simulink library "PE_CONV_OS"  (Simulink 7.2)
settings: Solver=ode45  SolverMode=SingleTasking  StartTime=0.0  StopTime=10.0  RelTol=1e-3
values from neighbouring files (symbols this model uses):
  C = 10e-3*1    (= 0.01)    [INIT_B6_2L_3Ph_IGBT_OS.m]    (also in INIT_B6_3L_3Ph_IGBT_OS.m; INIT_MMC_100L.m = 0.005; INIT_MMC_200L.m = 0.005; INIT_MMC_20L.m)
  FS = 900    [INIT_B6_2L_3Ph_IGBT_OS.m]    (also in INIT_B6_3L_3Ph_IGBT_OS.m; INIT_PWM_2L.m = 1000; INIT_PWM_3L.m = 1000; INIT_PWM_Con.m = 1000)
  LN = 2e-3    (= 0.002)    [INIT_PWM_2L.m]    (also in INIT_PWM_3L.m; INIT_PWM_Con.m; INIT_MMC_100L.m = 0.025; INIT_MMC_200L.m = 0.025)
  LS = 1e-3    (= 0.001)    [INIT_B6_2L_3Ph_IGBT_OS.m]    (also in INIT_B6_3L_3Ph_IGBT_OS.m; INIT_MMC_100L.m = 0.025; INIT_MMC_200L.m = 0.025; INIT_MMC_20L.m = 0.0025)
  LT = LN    (= 0.025)    [INIT_MMC_100L.m]    (also in INIT_MMC_200L.m; INIT_MMC_20L.m = 0.002; INIT_MMC_400L.m)
  Nc = 100    [INIT_MMC_100L.m]    (also in INIT_MMC_200L.m = 200; INIT_MMC_20L.m = 20; INIT_MMC_400L.m = 400)
  NT = sqrt(3)*340/400    [INIT_MMC_100L.m]    (also in INIT_MMC_200L.m; INIT_MMC_20L.m = sqrt(3); INIT_MMC_400L.m)
  Rg = 1e-3    (= 0.001)    [INIT_MMC_100L.m]    (also in INIT_MMC_200L.m; INIT_MMC_20L.m; INIT_MMC_400L.m)
  RN = 0.1    [INIT_PWM_2L.m]    (also in INIT_PWM_3L.m; INIT_PWM_Con.m; INIT_MMC_100L.m; INIT_MMC_200L.m)
  RT = RN    (= 0.1)    [INIT_MMC_100L.m]    (also in INIT_MMC_200L.m; INIT_MMC_20L.m; INIT_MMC_400L.m)
  UC0 = 600    [INIT_B6_2L_3Ph_IGBT_OS.m]    (also in INIT_B6_3L_3Ph_IGBT_OS.m = 500; INIT_MMC_100L.m = 6800; INIT_MMC_200L.m = 3400; INIT_MMC_20L.m = 5000)
undefined symbols (not defined in the file or in its folder): A, DT, FT, L, O1, O2, PHT, T, Td
libraries: simulink_extras x2
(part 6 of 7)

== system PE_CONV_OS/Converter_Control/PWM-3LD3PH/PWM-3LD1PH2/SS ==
  I1 : Inport  OutDataType=sfix(16)  OutScaling=2^0
  DT : DataTypeConversion
  DT1 : DataTypeConversion
  Relay : Relay  OutDataType=sfix(16)  OutScaling=2^0
  Sum : Sum  Inputs=+-  OutDataType=sfix(16)  OutScaling=2^0
  TonDelay : Subsystem  mask(TonDelay){DT=DT}
      mask prompts: DT "Dead Time"
      mask help: Turn on dead time to protect against short circuit of the converter leg
  TonDelay1 : Subsystem  mask(TonDelay){DT=DT}
      mask prompts: DT "Dead Time"
      mask help: Turn on dead time to protect against short circuit of the converter leg
  TriGtr-AO : Subsystem  mask(TriGtr-AO){A=A, O=O1, T=1/FT, Td=PHT/FT/180}
      mask prompts: A "Amplitude"; O "Offset"; T "Period Time"; Td "Time Delay"
      mask help: Triangular Wave Generator with variable time delay, variable amplitude and offset
  not : Logic  Operator=NOT  Inputs=1
  O1 : Outport  InitialOutput=0
  O2 : Outport  Port=2  InitialOutput=0
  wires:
  DT1/1 -> not/1
  DT/1 -> TonDelay1/1(s1)
  I1/1 -> Sum/1
  TriGtr-AO/1(Out1) -> Sum/2
  Sum/1 -> Relay/1
  not/1 -> DT/1
  TonDelay1/1(s1d) -> O2/1
  Relay/1 -> DT1/1, TonDelay/1(s1)
  TonDelay/1(s1d) -> O1/1

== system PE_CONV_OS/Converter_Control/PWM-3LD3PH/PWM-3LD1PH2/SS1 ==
  I1 : Inport  OutDataType=sfix(16)  OutScaling=2^0
  DT : DataTypeConversion
  DT1 : DataTypeConversion
  Relay : Relay  OutDataType=sfix(16)  OutScaling=2^0
  Sum : Sum  Inputs=+-  OutDataType=sfix(16)  OutScaling=2^0
  TonDelay : Subsystem  mask(TonDelay){DT=DT}
      mask prompts: DT "Dead Time"
      mask help: Turn on dead time to protect against short circuit of the converter leg
  TonDelay1 : Subsystem  mask(TonDelay){DT=DT}
      mask prompts: DT "Dead Time"
      mask help: Turn on dead time to protect against short circuit of the converter leg
  TriGtr-AO : Subsystem  mask(TriGtr-AO){A=A, O=O2, T=1/FT, Td=PHT/FT/180}
      mask prompts: A "Amplitude"; O "Offset"; T "Period Time"; Td "Time Delay"
      mask help: Triangular Wave Generator with variable time delay, variable amplitude and offset
  not : Logic  Operator=NOT  Inputs=1
  O1 : Outport  InitialOutput=0
  O2 : Outport  Port=2  InitialOutput=0
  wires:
  DT1/1 -> not/1
  DT/1 -> TonDelay1/1(s1)
  I1/1 -> Sum/1
  TriGtr-AO/1(Out1) -> Sum/2
  Sum/1 -> Relay/1
  not/1 -> DT/1
  TonDelay1/1(s1d) -> O2/1
  Relay/1 -> DT1/1, TonDelay/1(s1)
  TonDelay/1(s1d) -> O1/1

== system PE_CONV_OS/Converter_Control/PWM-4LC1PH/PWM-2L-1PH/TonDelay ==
  s1 : Inport  Orientation=down  OutDataType=sfix(16)  OutScaling=2^0
  Int : Integrator  ExternalReset=falling
  Rel1 : Relay  OnSwitchValue=DT  OutDataType=sfix(16)  OutScaling=2^0
  s1d : Outport  InitialOutput=0
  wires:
  Rel1/1 -> s1d/1
  s1/1 -> Int/1, Int/2
  Int/1 -> Rel1/1

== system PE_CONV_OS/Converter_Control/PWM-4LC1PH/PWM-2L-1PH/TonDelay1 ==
  s1 : Inport  Orientation=down  OutDataType=sfix(16)  OutScaling=2^0
  Int : Integrator  ExternalReset=falling
  Rel1 : Relay  OnSwitchValue=DT  OutDataType=sfix(16)  OutScaling=2^0
  s1d : Outport  InitialOutput=0
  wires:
  Rel1/1 -> s1d/1
  s1/1 -> Int/1, Int/2
  Int/1 -> Rel1/1

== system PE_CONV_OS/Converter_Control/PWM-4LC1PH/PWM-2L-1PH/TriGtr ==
  Clock : Clock
  S1 : Subsystem
  Sum : Sum  OutDataType=sfix(16)  OutScaling=2^0
  T : Constant  Value=T  OutDataType=sfix(16)  OutScaling=2^0
  Td : Constant  Value=Td  OutDataType=sfix(16)  OutScaling=2^0
  mod : Math  Operator=mod
  O : Outport  InitialOutput=0
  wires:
  Td/1 -> Sum/2
  Sum/1 -> mod/1
  T/1 -> mod/2
  Clock/1 -> Sum/1
  S1/1(Out1) -> O/1
  mod/1 -> S1/1(In1)

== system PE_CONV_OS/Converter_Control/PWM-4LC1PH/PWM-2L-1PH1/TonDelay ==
  s1 : Inport  Orientation=down  OutDataType=sfix(16)  OutScaling=2^0
  Int : Integrator  ExternalReset=falling
  Rel1 : Relay  OnSwitchValue=DT  OutDataType=sfix(16)  OutScaling=2^0
  s1d : Outport  InitialOutput=0
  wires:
  Int/1 -> Rel1/1
  s1/1 -> Int/2, Int/1
  Rel1/1 -> s1d/1

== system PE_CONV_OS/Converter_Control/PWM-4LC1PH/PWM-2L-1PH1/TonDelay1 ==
  s1 : Inport  Orientation=down  OutDataType=sfix(16)  OutScaling=2^0
  Int : Integrator  ExternalReset=falling
  Rel1 : Relay  OnSwitchValue=DT  OutDataType=sfix(16)  OutScaling=2^0
  s1d : Outport  InitialOutput=0
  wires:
  Int/1 -> Rel1/1
  s1/1 -> Int/2, Int/1
  Rel1/1 -> s1d/1

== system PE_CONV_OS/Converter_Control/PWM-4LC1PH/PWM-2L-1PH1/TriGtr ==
  Clock : Clock
  S1 : Subsystem
  Sum : Sum  OutDataType=sfix(16)  OutScaling=2^0
  T : Constant  Value=T  OutDataType=sfix(16)  OutScaling=2^0
  Td : Constant  Value=Td  OutDataType=sfix(16)  OutScaling=2^0
  mod : Math  Operator=mod
  O : Outport  InitialOutput=0
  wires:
  mod/1 -> S1/1(In1)
  S1/1(Out1) -> O/1
  Clock/1 -> Sum/1
  T/1 -> mod/2
  Sum/1 -> mod/1
  Td/1 -> Sum/2

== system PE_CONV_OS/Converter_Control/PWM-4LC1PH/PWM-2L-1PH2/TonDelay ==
  s1 : Inport  Orientation=down  OutDataType=sfix(16)  OutScaling=2^0
  Int : Integrator  ExternalReset=falling
  Rel1 : Relay  OnSwitchValue=DT  OutDataType=sfix(16)  OutScaling=2^0
  s1d : Outport  InitialOutput=0
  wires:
  Rel1/1 -> s1d/1
  s1/1 -> Int/1, Int/2
  Int/1 -> Rel1/1

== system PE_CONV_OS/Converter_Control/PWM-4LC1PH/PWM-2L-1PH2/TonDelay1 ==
  s1 : Inport  Orientation=down  OutDataType=sfix(16)  OutScaling=2^0
  Int : Integrator  ExternalReset=falling
  Rel1 : Relay  OnSwitchValue=DT  OutDataType=sfix(16)  OutScaling=2^0
  s1d : Outport  InitialOutput=0
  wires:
  Rel1/1 -> s1d/1
  s1/1 -> Int/1, Int/2
  Int/1 -> Rel1/1

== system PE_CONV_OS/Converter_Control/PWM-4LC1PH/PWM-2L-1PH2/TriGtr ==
  Clock : Clock
  S1 : Subsystem
  Sum : Sum  OutDataType=sfix(16)  OutScaling=2^0
  T : Constant  Value=T  OutDataType=sfix(16)  OutScaling=2^0
  Td : Constant  Value=Td  OutDataType=sfix(16)  OutScaling=2^0
  mod : Math  Operator=mod
  O : Outport  InitialOutput=0
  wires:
  Td/1 -> Sum/2
  Sum/1 -> mod/1
  T/1 -> mod/2
  Clock/1 -> Sum/1
  S1/1(Out1) -> O/1
  mod/1 -> S1/1(In1)

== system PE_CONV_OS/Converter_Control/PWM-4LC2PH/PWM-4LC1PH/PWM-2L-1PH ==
  In1 : Inport  OutDataType=sfix(16)  OutScaling=2^0
  DT : DataTypeConversion
  DT1 : DataTypeConversion
  Relay : Relay  OutDataType=sfix(16)  OutScaling=2^0
  Sum : Sum  Inputs=+-  OutDataType=sfix(16)  OutScaling=2^0
  TonDelay : Subsystem  mask(TonDelay){DT=DT}
      mask prompts: DT "Dead Time"
      mask help: Turn on dead time to protect against short circuit of the converter leg
  TonDelay1 : Subsystem  mask(TonDelay){DT=DT}
      mask prompts: DT "Dead Time"
      mask help: Turn on dead time to protect against short circuit of the converter leg
  TriGtr : Subsystem  mask(TriGtr){T=1/FT, Td=PHT/FT/360}
      mask prompts: T "Period Time"; Td "Time Delay"
      mask help: Triangular Wave Generator with variable time delay
  not : Logic  Operator=NOT  Inputs=1
  Out1 : Outport  InitialOutput=0
  Out2 : Outport  Port=2  InitialOutput=0
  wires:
  TonDelay/1(s1d) -> Out1/1
  Relay/1 -> TonDelay/1(s1), DT1/1
  TonDelay1/1(s1d) -> Out2/1
  not/1 -> DT/1
  Sum/1 -> Relay/1
  TriGtr/1(O) -> Sum/2
  In1/1 -> Sum/1
  DT/1 -> TonDelay1/1(s1)
  DT1/1 -> not/1

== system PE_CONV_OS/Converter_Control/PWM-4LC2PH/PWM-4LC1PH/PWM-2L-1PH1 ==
  In1 : Inport  OutDataType=sfix(16)  OutScaling=2^0
  DT : DataTypeConversion
  DT1 : DataTypeConversion
  Relay : Relay  OutDataType=sfix(16)  OutScaling=2^0
  Sum : Sum  Inputs=+-  OutDataType=sfix(16)  OutScaling=2^0
  TonDelay : Subsystem  mask(TonDelay){DT=DT}
      mask prompts: DT "Dead Time"
      mask help: Turn on dead time to protect against short circuit of the converter leg
  TonDelay1 : Subsystem  mask(TonDelay){DT=DT}
      mask prompts: DT "Dead Time"
      mask help: Turn on dead time to protect against short circuit of the converter leg
  TriGtr : Subsystem  mask(TriGtr){T=1/FT, Td=PHT/FT/360}
      mask prompts: T "Period Time"; Td "Time Delay"
      mask help: Triangular Wave Generator with variable time delay
  not : Logic  Operator=NOT  Inputs=1
  Out1 : Outport  InitialOutput=0
  Out2 : Outport  Port=2  InitialOutput=0
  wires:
  DT1/1 -> not/1
  DT/1 -> TonDelay1/1(s1)
  In1/1 -> Sum/1
  TriGtr/1(O) -> Sum/2
  Sum/1 -> Relay/1
  not/1 -> DT/1
  TonDelay1/1(s1d) -> Out2/1
  Relay/1 -> DT1/1, TonDelay/1(s1)
  TonDelay/1(s1d) -> Out1/1

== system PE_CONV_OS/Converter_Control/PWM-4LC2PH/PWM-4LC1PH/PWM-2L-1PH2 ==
  In1 : Inport  OutDataType=sfix(16)  OutScaling=2^0
  DT : DataTypeConversion
  DT1 : DataTypeConversion
  Relay : Relay  OutDataType=sfix(16)  OutScaling=2^0
  Sum : Sum  Inputs=+-  OutDataType=sfix(16)  OutScaling=2^0
  TonDelay : Subsystem  mask(TonDelay){DT=DT}
      mask prompts: DT "Dead Time"
      mask help: Turn on dead time to protect against short circuit of the converter leg
  TonDelay1 : Subsystem  mask(TonDelay){DT=DT}
      mask prompts: DT "Dead Time"
      mask help: Turn on dead time to protect against short circuit of the converter leg
  TriGtr : Subsystem  mask(TriGtr){T=1/FT, Td=PHT/FT/360}
      mask prompts: T "Period Time"; Td "Time Delay"
      mask help: Triangular Wave Generator with variable time delay
  not : Logic  Operator=NOT  Inputs=1
  Out1 : Outport  InitialOutput=0
  Out2 : Outport  Port=2  InitialOutput=0
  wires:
  TonDelay/1(s1d) -> Out1/1
  Relay/1 -> TonDelay/1(s1), DT1/1
  TonDelay1/1(s1d) -> Out2/1
  not/1 -> DT/1
  Sum/1 -> Relay/1
  TriGtr/1(O) -> Sum/2
  In1/1 -> Sum/1
  DT/1 -> TonDelay1/1(s1)
  DT1/1 -> not/1

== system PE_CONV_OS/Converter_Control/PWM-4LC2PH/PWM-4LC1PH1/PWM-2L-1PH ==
  In1 : Inport  OutDataType=sfix(16)  OutScaling=2^0
  DT : DataTypeConversion
  DT1 : DataTypeConversion
  Relay : Relay  OutDataType=sfix(16)  OutScaling=2^0
  Sum : Sum  Inputs=+-  OutDataType=sfix(16)  OutScaling=2^0
  TonDelay : Subsystem  mask(TonDelay){DT=DT}
      mask prompts: DT "Dead Time"
      mask help: Turn on dead time to protect against short circuit of the converter leg
  TonDelay1 : Subsystem  mask(TonDelay){DT=DT}
      mask prompts: DT "Dead Time"
      mask help: Turn on dead time to protect against short circuit of the converter leg
  TriGtr : Subsystem  mask(TriGtr){T=1/FT, Td=PHT/FT/360}
      mask prompts: T "Period Time"; Td "Time Delay"
      mask help: Triangular Wave Generator with variable time delay
  not : Logic  Operator=NOT  Inputs=1
  Out1 : Outport  InitialOutput=0
  Out2 : Outport  Port=2  InitialOutput=0
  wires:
  DT1/1 -> not/1
  DT/1 -> TonDelay1/1(s1)
  In1/1 -> Sum/1
  TriGtr/1(O) -> Sum/2
  Sum/1 -> Relay/1
  not/1 -> DT/1
  TonDelay1/1(s1d) -> Out2/1
  Relay/1 -> DT1/1, TonDelay/1(s1)
  TonDelay/1(s1d) -> Out1/1

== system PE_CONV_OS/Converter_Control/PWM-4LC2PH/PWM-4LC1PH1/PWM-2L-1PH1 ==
  In1 : Inport  OutDataType=sfix(16)  OutScaling=2^0
  DT : DataTypeConversion
  DT1 : DataTypeConversion
  Relay : Relay  OutDataType=sfix(16)  OutScaling=2^0
  Sum : Sum  Inputs=+-  OutDataType=sfix(16)  OutScaling=2^0
  TonDelay : Subsystem  mask(TonDelay){DT=DT}
      mask prompts: DT "Dead Time"
      mask help: Turn on dead time to protect against short circuit of the converter leg
  TonDelay1 : Subsystem  mask(TonDelay){DT=DT}
      mask prompts: DT "Dead Time"
      mask help: Turn on dead time to protect against short circuit of the converter leg
  TriGtr : Subsystem  mask(TriGtr){T=1/FT, Td=PHT/FT/360}
      mask prompts: T "Period Time"; Td "Time Delay"
      mask help: Triangular Wave Generator with variable time delay
  not : Logic  Operator=NOT  Inputs=1
  Out1 : Outport  InitialOutput=0
  Out2 : Outport  Port=2  InitialOutput=0
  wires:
  TonDelay/1(s1d) -> Out1/1
  Relay/1 -> TonDelay/1(s1), DT1/1
  TonDelay1/1(s1d) -> Out2/1
  not/1 -> DT/1
  Sum/1 -> Relay/1
  TriGtr/1(O) -> Sum/2
  In1/1 -> Sum/1
  DT/1 -> TonDelay1/1(s1)
  DT1/1 -> not/1

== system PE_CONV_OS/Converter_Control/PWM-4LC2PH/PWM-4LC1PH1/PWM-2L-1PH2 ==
  In1 : Inport  OutDataType=sfix(16)  OutScaling=2^0
  DT : DataTypeConversion
  DT1 : DataTypeConversion
  Relay : Relay  OutDataType=sfix(16)  OutScaling=2^0
  Sum : Sum  Inputs=+-  OutDataType=sfix(16)  OutScaling=2^0
  TonDelay : Subsystem  mask(TonDelay){DT=DT}
      mask prompts: DT "Dead Time"
      mask help: Turn on dead time to protect against short circuit of the converter leg
  TonDelay1 : Subsystem  mask(TonDelay){DT=DT}
      mask prompts: DT "Dead Time"
      mask help: Turn on dead time to protect against short circuit of the converter leg
  TriGtr : Subsystem  mask(TriGtr){T=1/FT, Td=PHT/FT/360}
      mask prompts: T "Period Time"; Td "Time Delay"
      mask help: Triangular Wave Generator with variable time delay
  not : Logic  Operator=NOT  Inputs=1
  Out1 : Outport  InitialOutput=0
  Out2 : Outport  Port=2  InitialOutput=0
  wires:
  DT1/1 -> not/1
  DT/1 -> TonDelay1/1(s1)
  In1/1 -> Sum/1
  TriGtr/1(O) -> Sum/2
  Sum/1 -> Relay/1
  not/1 -> DT/1
  TonDelay1/1(s1d) -> Out2/1
  Relay/1 -> DT1/1, TonDelay/1(s1)
  TonDelay/1(s1d) -> Out1/1

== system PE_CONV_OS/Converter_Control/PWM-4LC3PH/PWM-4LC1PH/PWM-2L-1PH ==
  In1 : Inport  OutDataType=sfix(16)  OutScaling=2^0
  DT : DataTypeConversion
  DT1 : DataTypeConversion
  Relay : Relay  OutDataType=sfix(16)  OutScaling=2^0
  Sum : Sum  Inputs=+-  OutDataType=sfix(16)  OutScaling=2^0
  TonDelay : Subsystem  mask(TonDelay){DT=DT}
      mask prompts: DT "Dead Time"
      mask help: Turn on dead time to protect against short circuit of the converter leg
  TonDelay1 : Subsystem  mask(TonDelay){DT=DT}
      mask prompts: DT "Dead Time"
      mask help: Turn on dead time to protect against short circuit of the converter leg
  TriGtr1 : Subsystem  mask(TriGtr){T=1/FT, Td=PHT/FT/360}
      mask prompts: T "Period Time"; Td "Time Delay"
      mask help: Triangular Wave Generator with variable time delay
  not : Logic  Operator=NOT  Inputs=1
  Out1 : Outport  InitialOutput=0
  Out2 : Outport  Port=2  InitialOutput=0
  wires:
  TonDelay/1(s1d) -> Out1/1
  Relay/1 -> TonDelay/1(s1), DT1/1
  TonDelay1/1(s1d) -> Out2/1
  not/1 -> DT/1
  Sum/1 -> Relay/1
  TriGtr1/1(O) -> Sum/2
  In1/1 -> Sum/1
  DT/1 -> TonDelay1/1(s1)
  DT1/1 -> not/1

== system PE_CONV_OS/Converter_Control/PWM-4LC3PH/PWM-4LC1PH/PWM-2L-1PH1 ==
  In1 : Inport  OutDataType=sfix(16)  OutScaling=2^0
  DT : DataTypeConversion
  DT1 : DataTypeConversion
  Relay : Relay  OutDataType=sfix(16)  OutScaling=2^0
  Sum : Sum  Inputs=+-  OutDataType=sfix(16)  OutScaling=2^0
  TonDelay : Subsystem  mask(TonDelay){DT=DT}
      mask prompts: DT "Dead Time"
      mask help: Turn on dead time to protect against short circuit of the converter leg
  TonDelay1 : Subsystem  mask(TonDelay){DT=DT}
      mask prompts: DT "Dead Time"
      mask help: Turn on dead time to protect against short circuit of the converter leg
  TriGtr1 : Subsystem  mask(TriGtr){T=1/FT, Td=PHT/FT/360}
      mask prompts: T "Period Time"; Td "Time Delay"
      mask help: Triangular Wave Generator with variable time delay
  not : Logic  Operator=NOT  Inputs=1
  Out1 : Outport  InitialOutput=0
  Out2 : Outport  Port=2  InitialOutput=0
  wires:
  DT1/1 -> not/1
  DT/1 -> TonDelay1/1(s1)
  In1/1 -> Sum/1
  TriGtr1/1(O) -> Sum/2
  Sum/1 -> Relay/1
  not/1 -> DT/1
  TonDelay1/1(s1d) -> Out2/1
  Relay/1 -> DT1/1, TonDelay/1(s1)
  TonDelay/1(s1d) -> Out1/1

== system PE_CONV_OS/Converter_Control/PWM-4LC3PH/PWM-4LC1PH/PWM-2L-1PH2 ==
  In1 : Inport  OutDataType=sfix(16)  OutScaling=2^0
  DT : DataTypeConversion
  DT1 : DataTypeConversion
  Relay : Relay  OutDataType=sfix(16)  OutScaling=2^0
  Sum : Sum  Inputs=+-  OutDataType=sfix(16)  OutScaling=2^0
  TonDelay : Subsystem  mask(TonDelay){DT=DT}
      mask prompts: DT "Dead Time"
      mask help: Turn on dead time to protect against short circuit of the converter leg
  TonDelay1 : Subsystem  mask(TonDelay){DT=DT}
      mask prompts: DT "Dead Time"
      mask help: Turn on dead time to protect against short circuit of the converter leg
  TriGtr1 : Subsystem  mask(TriGtr){T=1/FT, Td=PHT/FT/360}
      mask prompts: T "Period Time"; Td "Time Delay"
      mask help: Triangular Wave Generator with variable time delay
  not : Logic  Operator=NOT  Inputs=1
  Out1 : Outport  InitialOutput=0
  Out2 : Outport  Port=2  InitialOutput=0
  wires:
  TonDelay/1(s1d) -> Out1/1
  Relay/1 -> TonDelay/1(s1), DT1/1
  TonDelay1/1(s1d) -> Out2/1
  not/1 -> DT/1
  Sum/1 -> Relay/1
  TriGtr1/1(O) -> Sum/2
  In1/1 -> Sum/1
  DT/1 -> TonDelay1/1(s1)
  DT1/1 -> not/1

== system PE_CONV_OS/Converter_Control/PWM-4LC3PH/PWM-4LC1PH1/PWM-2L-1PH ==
  In1 : Inport  OutDataType=sfix(16)  OutScaling=2^0
  DT : DataTypeConversion
  DT1 : DataTypeConversion
  Relay : Relay  OutDataType=sfix(16)  OutScaling=2^0
  Sum : Sum  Inputs=+-  OutDataType=sfix(16)  OutScaling=2^0
  TonDelay : Subsystem  mask(TonDelay){DT=DT}
      mask prompts: DT "Dead Time"
      mask help: Turn on dead time to protect against short circuit of the converter leg
  TonDelay1 : Subsystem  mask(TonDelay){DT=DT}
      mask prompts: DT "Dead Time"
      mask help: Turn on dead time to protect against short circuit of the converter leg
  TriGtr1 : Subsystem  mask(TriGtr){T=1/FT, Td=PHT/FT/360}
      mask prompts: T "Period Time"; Td "Time Delay"
      mask help: Triangular Wave Generator with variable time delay
  not : Logic  Operator=NOT  Inputs=1
  Out1 : Outport  InitialOutput=0
  Out2 : Outport  Port=2  InitialOutput=0
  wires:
  DT1/1 -> not/1
  DT/1 -> TonDelay1/1(s1)
  In1/1 -> Sum/1
  TriGtr1/1(O) -> Sum/2
  Sum/1 -> Relay/1
  not/1 -> DT/1
  TonDelay1/1(s1d) -> Out2/1
  Relay/1 -> DT1/1, TonDelay/1(s1)
  TonDelay/1(s1d) -> Out1/1

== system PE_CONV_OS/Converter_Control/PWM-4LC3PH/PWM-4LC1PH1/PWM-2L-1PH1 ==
  In1 : Inport  OutDataType=sfix(16)  OutScaling=2^0
  DT : DataTypeConversion
  DT1 : DataTypeConversion
  Relay : Relay  OutDataType=sfix(16)  OutScaling=2^0
  Sum : Sum  Inputs=+-  OutDataType=sfix(16)  OutScaling=2^0
  TonDelay : Subsystem  mask(TonDelay){DT=DT}
      mask prompts: DT "Dead Time"
      mask help: Turn on dead time to protect against short circuit of the converter leg
  TonDelay1 : Subsystem  mask(TonDelay){DT=DT}
      mask prompts: DT "Dead Time"
      mask help: Turn on dead time to protect against short circuit of the converter leg
  TriGtr1 : Subsystem  mask(TriGtr){T=1/FT, Td=PHT/FT/360}
      mask prompts: T "Period Time"; Td "Time Delay"
      mask help: Triangular Wave Generator with variable time delay
  not : Logic  Operator=NOT  Inputs=1
  Out1 : Outport  InitialOutput=0
  Out2 : Outport  Port=2  InitialOutput=0
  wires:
  TonDelay/1(s1d) -> Out1/1
  Relay/1 -> TonDelay/1(s1), DT1/1
  TonDelay1/1(s1d) -> Out2/1
  not/1 -> DT/1
  Sum/1 -> Relay/1
  TriGtr1/1(O) -> Sum/2
  In1/1 -> Sum/1
  DT/1 -> TonDelay1/1(s1)
  DT1/1 -> not/1

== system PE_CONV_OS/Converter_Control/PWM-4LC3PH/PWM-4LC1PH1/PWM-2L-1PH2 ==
  In1 : Inport  OutDataType=sfix(16)  OutScaling=2^0
  DT : DataTypeConversion
  DT1 : DataTypeConversion
  Relay : Relay  OutDataType=sfix(16)  OutScaling=2^0
  Sum : Sum  Inputs=+-  OutDataType=sfix(16)  OutScaling=2^0
  TonDelay : Subsystem  mask(TonDelay){DT=DT}
      mask prompts: DT "Dead Time"
      mask help: Turn on dead time to protect against short circuit of the converter leg
  TonDelay1 : Subsystem  mask(TonDelay){DT=DT}
      mask prompts: DT "Dead Time"
      mask help: Turn on dead time to protect against short circuit of the converter leg
  TriGtr1 : Subsystem  mask(TriGtr){T=1/FT, Td=PHT/FT/360}
      mask prompts: T "Period Time"; Td "Time Delay"
      mask help: Triangular Wave Generator with variable time delay
  not : Logic  Operator=NOT  Inputs=1
  Out1 : Outport  InitialOutput=0
  Out2 : Outport  Port=2  InitialOutput=0
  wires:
  DT1/1 -> not/1
  DT/1 -> TonDelay1/1(s1)
  In1/1 -> Sum/1
  TriGtr1/1(O) -> Sum/2
  Sum/1 -> Relay/1
  not/1 -> DT/1
  TonDelay1/1(s1d) -> Out2/1
  Relay/1 -> DT1/1, TonDelay/1(s1)
  TonDelay/1(s1d) -> Out1/1

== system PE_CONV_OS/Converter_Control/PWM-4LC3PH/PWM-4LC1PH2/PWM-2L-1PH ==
  In1 : Inport  OutDataType=sfix(16)  OutScaling=2^0
  DT : DataTypeConversion
  DT1 : DataTypeConversion
  Relay : Relay  OutDataType=sfix(16)  OutScaling=2^0
  Sum : Sum  Inputs=+-  OutDataType=sfix(16)  OutScaling=2^0
  TonDelay : Subsystem  mask(TonDelay){DT=DT}
      mask prompts: DT "Dead Time"
      mask help: Turn on dead time to protect against short circuit of the converter leg
  TonDelay1 : Subsystem  mask(TonDelay){DT=DT}
      mask prompts: DT "Dead Time"
      mask help: Turn on dead time to protect against short circuit of the converter leg
  TriGtr1 : Subsystem  mask(TriGtr){T=1/FT, Td=PHT/FT/360}
      mask prompts: T "Period Time"; Td "Time Delay"
      mask help: Triangular Wave Generator with variable time delay
  not : Logic  Operator=NOT  Inputs=1
  Out1 : Outport  InitialOutput=0
  Out2 : Outport  Port=2  InitialOutput=0
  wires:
  TonDelay/1(s1d) -> Out1/1
  Relay/1 -> TonDelay/1(s1), DT1/1
  TonDelay1/1(s1d) -> Out2/1
  not/1 -> DT/1
  Sum/1 -> Relay/1
  TriGtr1/1(O) -> Sum/2
  In1/1 -> Sum/1
  DT/1 -> TonDelay1/1(s1)
  DT1/1 -> not/1

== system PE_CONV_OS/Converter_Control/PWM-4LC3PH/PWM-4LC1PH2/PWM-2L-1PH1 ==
  In1 : Inport  OutDataType=sfix(16)  OutScaling=2^0
  DT : DataTypeConversion
  DT1 : DataTypeConversion
  Relay : Relay  OutDataType=sfix(16)  OutScaling=2^0
  Sum : Sum  Inputs=+-  OutDataType=sfix(16)  OutScaling=2^0
  TonDelay : Subsystem  mask(TonDelay){DT=DT}
      mask prompts: DT "Dead Time"
      mask help: Turn on dead time to protect against short circuit of the converter leg
  TonDelay1 : Subsystem  mask(TonDelay){DT=DT}
      mask prompts: DT "Dead Time"
      mask help: Turn on dead time to protect against short circuit of the converter leg
  TriGtr1 : Subsystem  mask(TriGtr){T=1/FT, Td=PHT/FT/360}
      mask prompts: T "Period Time"; Td "Time Delay"
      mask help: Triangular Wave Generator with variable time delay
  not : Logic  Operator=NOT  Inputs=1
  Out1 : Outport  InitialOutput=0
  Out2 : Outport  Port=2  InitialOutput=0
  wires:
  DT1/1 -> not/1
  DT/1 -> TonDelay1/1(s1)
  In1/1 -> Sum/1
  TriGtr1/1(O) -> Sum/2
  Sum/1 -> Relay/1
  not/1 -> DT/1
  TonDelay1/1(s1d) -> Out2/1
  Relay/1 -> DT1/1, TonDelay/1(s1)
  TonDelay/1(s1d) -> Out1/1

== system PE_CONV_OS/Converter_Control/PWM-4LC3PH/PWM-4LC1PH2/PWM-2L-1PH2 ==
  In1 : Inport  OutDataType=sfix(16)  OutScaling=2^0
  DT : DataTypeConversion
  DT1 : DataTypeConversion
  Relay : Relay  OutDataType=sfix(16)  OutScaling=2^0
  Sum : Sum  Inputs=+-  OutDataType=sfix(16)  OutScaling=2^0
  TonDelay : Subsystem  mask(TonDelay){DT=DT}
      mask prompts: DT "Dead Time"
      mask help: Turn on dead time to protect against short circuit of the converter leg
  TonDelay1 : Subsystem  mask(TonDelay){DT=DT}
      mask prompts: DT "Dead Time"
      mask help: Turn on dead time to protect against short circuit of the converter leg
  TriGtr1 : Subsystem  mask(TriGtr){T=1/FT, Td=PHT/FT/360}
      mask prompts: T "Period Time"; Td "Time Delay"
      mask help: Triangular Wave Generator with variable time delay
  not : Logic  Operator=NOT  Inputs=1
  Out1 : Outport  InitialOutput=0
  Out2 : Outport  Port=2  InitialOutput=0
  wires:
  TonDelay/1(s1d) -> Out1/1
  Relay/1 -> TonDelay/1(s1), DT1/1
  TonDelay1/1(s1d) -> Out2/1
  not/1 -> DT/1
  Sum/1 -> Relay/1
  TriGtr1/1(O) -> Sum/2
  In1/1 -> Sum/1
  DT/1 -> TonDelay1/1(s1)
  DT1/1 -> not/1

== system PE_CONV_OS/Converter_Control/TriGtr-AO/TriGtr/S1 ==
  I1 : Inport
  Fcn : Fcn  Expr="(u* (u <=T/4) * 4/T)   +  (  (u > T/4) && ( u <=3*T/4) )* ( 1 - (u-T/4) *4/T )   +  ( (u > 3*T/4)&& (u<=T)) * ( ((u -3*T/4)* 4/T )-1 )"
  O1 : Outport
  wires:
  Fcn/1 -> O1/1
  I1/1 -> Fcn/1

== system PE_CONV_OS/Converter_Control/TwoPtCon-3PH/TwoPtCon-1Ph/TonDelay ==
  s1 : Inport  Orientation=down  OutDataType=sfix(16)  OutScaling=2^0
  Int : Integrator  ExternalReset=falling
  Rel1 : Relay  OnSwitchValue=DT  OutDataType=sfix(16)  OutScaling=2^0
  s1d : Outport  InitialOutput=0
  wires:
  Rel1/1 -> s1d/1
  s1/1 -> Int/1, Int/2
  Int/1 -> Rel1/1

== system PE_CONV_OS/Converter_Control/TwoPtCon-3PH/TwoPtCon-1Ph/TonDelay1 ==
  s1 : Inport  Orientation=down  OutDataType=sfix(16)  OutScaling=2^0
  Int : Integrator  ExternalReset=falling
  Rel1 : Relay  OnSwitchValue=DT  OutDataType=sfix(16)  OutScaling=2^0
  s1d : Outport  InitialOutput=0
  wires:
  Rel1/1 -> s1d/1
  s1/1 -> Int/1, Int/2
  Int/1 -> Rel1/1

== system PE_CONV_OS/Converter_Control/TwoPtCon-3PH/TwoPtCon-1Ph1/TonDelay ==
  s1 : Inport  Orientation=down  OutDataType=sfix(16)  OutScaling=2^0
  Int : Integrator  ExternalReset=falling
  Rel1 : Relay  OnSwitchValue=DT  OutDataType=sfix(16)  OutScaling=2^0
  s1d : Outport  InitialOutput=0
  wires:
  Rel1/1 -> s1d/1
  s1/1 -> Int/1, Int/2
  Int/1 -> Rel1/1

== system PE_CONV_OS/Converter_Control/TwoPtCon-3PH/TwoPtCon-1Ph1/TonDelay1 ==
  s1 : Inport  Orientation=down  OutDataType=sfix(16)  OutScaling=2^0
  Int : Integrator  ExternalReset=falling
  Rel1 : Relay  OnSwitchValue=DT  OutDataType=sfix(16)  OutScaling=2^0
  s1d : Outport  InitialOutput=0
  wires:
  Rel1/1 -> s1d/1
  s1/1 -> Int/1, Int/2
  Int/1 -> Rel1/1

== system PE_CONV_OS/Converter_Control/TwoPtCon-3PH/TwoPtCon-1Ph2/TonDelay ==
  s1 : Inport  Orientation=down  OutDataType=sfix(16)  OutScaling=2^0
  Int : Integrator  ExternalReset=falling
  Rel1 : Relay  OnSwitchValue=DT  OutDataType=sfix(16)  OutScaling=2^0
  s1d : Outport  InitialOutput=0
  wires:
  Rel1/1 -> s1d/1
  s1/1 -> Int/1, Int/2
  Int/1 -> Rel1/1

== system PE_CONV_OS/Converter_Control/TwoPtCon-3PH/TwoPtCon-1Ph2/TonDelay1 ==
  s1 : Inport  Orientation=down  OutDataType=sfix(16)  OutScaling=2^0
  Int : Integrator  ExternalReset=falling
  Rel1 : Relay  OnSwitchValue=DT  OutDataType=sfix(16)  OutScaling=2^0
  s1d : Outport  InitialOutput=0
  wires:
  Rel1/1 -> s1d/1
  s1/1 -> Int/1, Int/2
  Int/1 -> Rel1/1

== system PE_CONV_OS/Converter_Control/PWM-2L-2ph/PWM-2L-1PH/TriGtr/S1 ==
  I1 : Inport  OutDataType=sfix(16)  OutScaling=2^0
  Fcn : Fcn  Expr=u* (u <=T/4) * 4/T
  Fcn1 : Fcn  Expr="(  (u > T/4) && ( u <=3*T/4) )* ( 1 - (u-T/4) *4/T )"
  Fcn2 : Fcn  Expr=( (u > 3*T/4)&& (u<=T)) * ( ((u -3*T/4)* 4/T )-1 )
  Sum1 : Sum  Inputs=+++  OutDataType=sfix(16)  OutScaling=2^0
  O1 : Outport
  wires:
  I1/1 -> Fcn1/1, Fcn2/1, Fcn/1
  Sum1/1 -> O1/1
  Fcn/1 -> Sum1/1
  Fcn1/1 -> Sum1/2
  Fcn2/1 -> Sum1/3

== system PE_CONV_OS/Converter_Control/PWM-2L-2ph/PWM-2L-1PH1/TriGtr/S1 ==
  I1 : Inport  OutDataType=sfix(16)  OutScaling=2^0
  Fcn : Fcn  Expr=u* (u <=T/4) * 4/T
  Fcn1 : Fcn  Expr="(  (u > T/4) && ( u <=3*T/4) )* ( 1 - (u-T/4) *4/T )"
  Fcn2 : Fcn  Expr=( (u > 3*T/4)&& (u<=T)) * ( ((u -3*T/4)* 4/T )-1 )
  Sum1 : Sum  Inputs=+++  OutDataType=sfix(16)  OutScaling=2^0
  O1 : Outport
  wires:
  Fcn2/1 -> Sum1/3
  Fcn1/1 -> Sum1/2
  Fcn/1 -> Sum1/1
  Sum1/1 -> O1/1
  I1/1 -> Fcn/1, Fcn2/1, Fcn1/1

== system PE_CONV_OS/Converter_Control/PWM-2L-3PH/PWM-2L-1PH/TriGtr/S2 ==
  I1 : Inport
  Fcn : Fcn  Expr="(u* (u <=T/4) * 4/T)   +  (  (u > T/4) && ( u <=3*T/4) )* ( 1 - (u-T/4) *4/T )   +  ( (u > 3*T/4)&& (u<=T)) * ( ((u -3*T/4)* 4/T )-1 )"
  O1 : Outport
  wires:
  Fcn/1 -> O1/1
  I1/1 -> Fcn/1

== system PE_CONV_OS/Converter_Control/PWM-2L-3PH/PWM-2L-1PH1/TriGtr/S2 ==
  I1 : Inport
  Fcn : Fcn  Expr="(u* (u <=T/4) * 4/T)   +  (  (u > T/4) && ( u <=3*T/4) )* ( 1 - (u-T/4) *4/T )   +  ( (u > 3*T/4)&& (u<=T)) * ( ((u -3*T/4)* 4/T )-1 )"
  O1 : Outport
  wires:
  I1/1 -> Fcn/1
  Fcn/1 -> O1/1

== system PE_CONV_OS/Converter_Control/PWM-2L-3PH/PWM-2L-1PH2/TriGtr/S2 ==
  I1 : Inport
  Fcn : Fcn  Expr="(u* (u <=T/4) * 4/T)   +  (  (u > T/4) && ( u <=3*T/4) )* ( 1 - (u-T/4) *4/T )   +  ( (u > 3*T/4)&& (u<=T)) * ( ((u -3*T/4)* 4/T )-1 )"
  O1 : Outport
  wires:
  Fcn/1 -> O1/1
  I1/1 -> Fcn/1

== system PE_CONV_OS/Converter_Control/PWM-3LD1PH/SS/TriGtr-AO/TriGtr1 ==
  Clock : Clock
  S2 : Subsystem
  Sum : Sum  OutDataType=sfix(16)  OutScaling=2^0
  T : Constant  Value=T  OutDataType=sfix(16)  OutScaling=2^0
  Td : Constant  Value=Td  OutDataType=sfix(16)  OutScaling=2^0
  mod : Math  Operator=mod
  O : Outport  InitialOutput=0
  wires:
  Td/1 -> Sum/2
  Sum/1 -> mod/1
  T/1 -> mod/2
  Clock/1 -> Sum/1
  S2/1(O1) -> O/1
  mod/1 -> S2/1(I1)

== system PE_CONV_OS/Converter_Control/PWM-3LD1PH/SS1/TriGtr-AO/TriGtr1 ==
  Clock : Clock
  S1 : Subsystem
  Sum : Sum
  T : Constant  Value=T
  Td : Constant  Value=Td
  mod : Math  Operator=mod
  O : Outport  InitialOutput=0
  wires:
  Td/1 -> Sum/2
  Sum/1 -> mod/1
  T/1 -> mod/2
  Clock/1 -> Sum/1
  S1/1(O1) -> O/1
  mod/1 -> S1/1(I1)

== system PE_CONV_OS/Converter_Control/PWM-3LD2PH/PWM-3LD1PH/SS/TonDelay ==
  s1 : Inport  Orientation=down  OutDataType=sfix(16)  OutScaling=2^0
  Int : Integrator  ExternalReset=falling
  Rel1 : Relay  OnSwitchValue=DT  OutDataType=sfix(16)  OutScaling=2^0
  s1d : Outport  InitialOutput=0
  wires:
  Int/1 -> Rel1/1
  s1/1 -> Int/2, Int/1
  Rel1/1 -> s1d/1

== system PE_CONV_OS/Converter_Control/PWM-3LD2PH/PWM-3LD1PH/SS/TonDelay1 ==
  s1 : Inport  Orientation=down  OutDataType=sfix(16)  OutScaling=2^0
  Int : Integrator  ExternalReset=falling
  Rel1 : Relay  OnSwitchValue=DT  OutDataType=sfix(16)  OutScaling=2^0
  s1d : Outport  InitialOutput=0
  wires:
  Int/1 -> Rel1/1
  s1/1 -> Int/2, Int/1
  Rel1/1 -> s1d/1

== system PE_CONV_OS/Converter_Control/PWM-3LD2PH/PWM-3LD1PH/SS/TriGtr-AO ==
  Ampl. : Gain  Gain=A  ParameterDataType=sfix(16)  ParameterScaling=2^0  OutDataType=sfix(16)  OutScaling=2^0
  Offset : Constant  Value=O  OutDataType=sfix(16)  OutScaling=2^0
  Sum : Sum  OutDataType=sfix(16)  OutScaling=2^0
  TriGtr : Subsystem  mask(TriGtr){T=1/FT, Td=PHT/FT/180}
      mask prompts: T "Period Time"; Td "Time Delay"
      mask help: Triangular Wave Generator with variable time delay
  Out1 : Outport
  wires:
  Offset/1 -> Sum/2
  TriGtr/1(O) -> Ampl./1
  Ampl./1 -> Sum/1
  Sum/1 -> Out1/1

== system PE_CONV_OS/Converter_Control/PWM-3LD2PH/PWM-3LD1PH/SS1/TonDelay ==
  s1 : Inport  Orientation=down  OutDataType=sfix(16)  OutScaling=2^0
  Int : Integrator  ExternalReset=falling
  Rel1 : Relay  OnSwitchValue=DT  OutDataType=sfix(16)  OutScaling=2^0
  s1d : Outport  InitialOutput=0
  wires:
  Int/1 -> Rel1/1
  s1/1 -> Int/2, Int/1
  Rel1/1 -> s1d/1

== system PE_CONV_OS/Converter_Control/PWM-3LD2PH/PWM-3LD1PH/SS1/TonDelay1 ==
  s1 : Inport  Orientation=down  OutDataType=sfix(16)  OutScaling=2^0
  Int : Integrator  ExternalReset=falling
  Rel1 : Relay  OnSwitchValue=DT  OutDataType=sfix(16)  OutScaling=2^0
  s1d : Outport  InitialOutput=0
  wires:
  Int/1 -> Rel1/1
  s1/1 -> Int/2, Int/1
  Rel1/1 -> s1d/1

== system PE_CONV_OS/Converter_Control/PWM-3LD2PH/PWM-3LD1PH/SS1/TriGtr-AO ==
  Ampl. : Gain  Gain=A  ParameterDataType=sfix(16)  ParameterScaling=2^0  OutDataType=sfix(16)  OutScaling=2^0
  Offset : Constant  Value=O  OutDataType=sfix(16)  OutScaling=2^0
  Sum : Sum  OutDataType=sfix(16)  OutScaling=2^0
  TriGtr1 : Subsystem  mask(TriGtr){T=1/FT, Td=PHT/FT/180}
      mask prompts: T "Period Time"; Td "Time Delay"
      mask help: Triangular Wave Generator with variable time delay
  Out1 : Outport
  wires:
  Sum/1 -> Out1/1
  Ampl./1 -> Sum/1
  TriGtr1/1(O) -> Ampl./1
  Offset/1 -> Sum/2

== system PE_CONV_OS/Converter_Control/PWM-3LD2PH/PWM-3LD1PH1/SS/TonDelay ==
  s1 : Inport  Orientation=down  OutDataType=sfix(16)  OutScaling=2^0
  Int : Integrator  ExternalReset=falling
  Rel1 : Relay  OnSwitchValue=DT  OutDataType=sfix(16)  OutScaling=2^0
  s1d : Outport  InitialOutput=0
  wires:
  Rel1/1 -> s1d/1
  s1/1 -> Int/1, Int/2
  Int/1 -> Rel1/1

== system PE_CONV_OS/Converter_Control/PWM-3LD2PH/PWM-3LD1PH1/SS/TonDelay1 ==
  s1 : Inport  Orientation=down  OutDataType=sfix(16)  OutScaling=2^0
  Int : Integrator  ExternalReset=falling
  Rel1 : Relay  OnSwitchValue=DT  OutDataType=sfix(16)  OutScaling=2^0
  s1d : Outport  InitialOutput=0
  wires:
  Rel1/1 -> s1d/1
  s1/1 -> Int/1, Int/2
  Int/1 -> Rel1/1

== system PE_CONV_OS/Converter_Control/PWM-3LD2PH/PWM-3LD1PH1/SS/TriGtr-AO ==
  Ampl. : Gain  Gain=A  ParameterDataType=sfix(16)  ParameterScaling=2^0  OutDataType=sfix(16)  OutScaling=2^0
  Offset : Constant  Value=O  OutDataType=sfix(16)  OutScaling=2^0
  Sum : Sum  OutDataType=sfix(16)  OutScaling=2^0
  TriGtr : Subsystem  mask(TriGtr){T=1/FT, Td=PHT/FT/180}
      mask prompts: T "Period Time"; Td "Time Delay"
      mask help: Triangular Wave Generator with variable time delay
  Out1 : Outport
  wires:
  Sum/1 -> Out1/1
  Ampl./1 -> Sum/1
  TriGtr/1(O) -> Ampl./1
  Offset/1 -> Sum/2

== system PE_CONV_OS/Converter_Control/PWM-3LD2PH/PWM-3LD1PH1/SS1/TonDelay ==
  s1 : Inport  Orientation=down  OutDataType=sfix(16)  OutScaling=2^0
  Int : Integrator  ExternalReset=falling
  Rel1 : Relay  OnSwitchValue=DT  OutDataType=sfix(16)  OutScaling=2^0
  s1d : Outport  InitialOutput=0
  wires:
  Rel1/1 -> s1d/1
  s1/1 -> Int/1, Int/2
  Int/1 -> Rel1/1

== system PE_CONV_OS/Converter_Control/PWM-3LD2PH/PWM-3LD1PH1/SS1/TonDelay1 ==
  s1 : Inport  Orientation=down  OutDataType=sfix(16)  OutScaling=2^0
  Int : Integrator  ExternalReset=falling
  Rel1 : Relay  OnSwitchValue=DT  OutDataType=sfix(16)  OutScaling=2^0
  s1d : Outport  InitialOutput=0
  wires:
  Rel1/1 -> s1d/1
  s1/1 -> Int/1, Int/2
  Int/1 -> Rel1/1

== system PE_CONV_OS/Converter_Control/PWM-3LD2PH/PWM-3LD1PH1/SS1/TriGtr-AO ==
  Ampl. : Gain  Gain=A  ParameterDataType=sfix(16)  ParameterScaling=2^0  OutDataType=sfix(16)  OutScaling=2^0
  Offset : Constant  Value=O  OutDataType=sfix(16)  OutScaling=2^0
  Sum : Sum  OutDataType=sfix(16)  OutScaling=2^0
  TriGtr : Subsystem  mask(TriGtr){T=1/FT, Td=PHT/FT/180}
      mask prompts: T "Period Time"; Td "Time Delay"
      mask help: Triangular Wave Generator with variable time delay
  Out1 : Outport
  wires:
  Offset/1 -> Sum/2
  TriGtr/1(O) -> Ampl./1
  Ampl./1 -> Sum/1
  Sum/1 -> Out1/1

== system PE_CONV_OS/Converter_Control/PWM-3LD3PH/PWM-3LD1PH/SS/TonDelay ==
  s1 : Inport  Orientation=down  OutDataType=sfix(16)  OutScaling=2^0
  Int : Integrator  ExternalReset=falling
  Rel1 : Relay  OnSwitchValue=DT  OutDataType=sfix(16)  OutScaling=2^0
  s1d : Outport  InitialOutput=0
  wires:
  Int/1 -> Rel1/1
  s1/1 -> Int/2, Int/1
  Rel1/1 -> s1d/1

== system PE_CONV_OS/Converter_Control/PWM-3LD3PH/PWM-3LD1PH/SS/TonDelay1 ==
  s1 : Inport  Orientation=down  OutDataType=sfix(16)  OutScaling=2^0
  Int : Integrator  ExternalReset=falling
  Rel1 : Relay  OnSwitchValue=DT  OutDataType=sfix(16)  OutScaling=2^0
  s1d : Outport  InitialOutput=0
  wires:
  Int/1 -> Rel1/1
  s1/1 -> Int/2, Int/1
  Rel1/1 -> s1d/1

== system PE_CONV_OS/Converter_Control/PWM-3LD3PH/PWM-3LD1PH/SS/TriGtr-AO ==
  Ampl. : Gain  Gain=A  ParameterDataType=sfix(16)  ParameterScaling=2^0  OutDataType=sfix(16)  OutScaling=2^0
  Offset : Constant  Value=O  OutDataType=sfix(16)  OutScaling=2^0
  Sum : Sum  OutDataType=sfix(16)  OutScaling=2^0
  TriGtr1 : Subsystem  mask(TriGtr){T=T, Td=Td}
      mask prompts: T "Period Time"; Td "Time Delay"
      mask help: Triangular Wave Generator with variable time delay
  Out1 : Outport
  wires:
  Offset/1 -> Sum/2
  TriGtr1/1(O) -> Ampl./1
  Ampl./1 -> Sum/1
  Sum/1 -> Out1/1

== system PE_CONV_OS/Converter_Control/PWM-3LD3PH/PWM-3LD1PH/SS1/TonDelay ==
  s1 : Inport  Orientation=down  OutDataType=sfix(16)  OutScaling=2^0
  Int : Integrator  ExternalReset=falling
  Rel1 : Relay  OnSwitchValue=DT  OutDataType=sfix(16)  OutScaling=2^0
  s1d : Outport  InitialOutput=0
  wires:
  Int/1 -> Rel1/1
  s1/1 -> Int/2, Int/1
  Rel1/1 -> s1d/1

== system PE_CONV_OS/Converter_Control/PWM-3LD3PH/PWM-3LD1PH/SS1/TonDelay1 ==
  s1 : Inport  Orientation=down  OutDataType=sfix(16)  OutScaling=2^0
  Int : Integrator  ExternalReset=falling
  Rel1 : Relay  OnSwitchValue=DT  OutDataType=sfix(16)  OutScaling=2^0
  s1d : Outport  InitialOutput=0
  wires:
  Int/1 -> Rel1/1
  s1/1 -> Int/2, Int/1
  Rel1/1 -> s1d/1

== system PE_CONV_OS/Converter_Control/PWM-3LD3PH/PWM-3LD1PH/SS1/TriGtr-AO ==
  Ampl. : Gain  Gain=A  ParameterDataType=sfix(16)  ParameterScaling=2^0  OutDataType=sfix(16)  OutScaling=2^0
  Offset : Constant  Value=O  OutDataType=sfix(16)  OutScaling=2^0
  Sum : Sum  OutDataType=sfix(16)  OutScaling=2^0
  TriGtr1 : Subsystem  mask(TriGtr){T=T, Td=Td}
      mask prompts: T "Period Time"; Td "Time Delay"
      mask help: Triangular Wave Generator with variable time delay
  Out1 : Outport
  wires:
  Sum/1 -> Out1/1
  Ampl./1 -> Sum/1
  TriGtr1/1(O) -> Ampl./1
  Offset/1 -> Sum/2

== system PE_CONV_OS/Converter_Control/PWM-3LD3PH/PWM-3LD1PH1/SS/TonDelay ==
  s1 : Inport  Orientation=down  OutDataType=sfix(16)  OutScaling=2^0
  Int : Integrator  ExternalReset=falling
  Rel1 : Relay  OnSwitchValue=DT  OutDataType=sfix(16)  OutScaling=2^0
  s1d : Outport  InitialOutput=0
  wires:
  Rel1/1 -> s1d/1
  s1/1 -> Int/1, Int/2
  Int/1 -> Rel1/1

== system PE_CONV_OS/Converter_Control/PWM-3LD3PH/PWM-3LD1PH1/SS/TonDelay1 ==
  s1 : Inport  Orientation=down  OutDataType=sfix(16)  OutScaling=2^0
  Int : Integrator  ExternalReset=falling
  Rel1 : Relay  OnSwitchValue=DT  OutDataType=sfix(16)  OutScaling=2^0
  s1d : Outport  InitialOutput=0
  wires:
  Rel1/1 -> s1d/1
  s1/1 -> Int/1, Int/2
  Int/1 -> Rel1/1

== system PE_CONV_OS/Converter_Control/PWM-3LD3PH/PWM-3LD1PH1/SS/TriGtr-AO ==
  Ampl. : Gain  Gain=A  ParameterDataType=sfix(16)  ParameterScaling=2^0  OutDataType=sfix(16)  OutScaling=2^0
  Offset : Constant  Value=O  OutDataType=sfix(16)  OutScaling=2^0
  Sum : Sum  OutDataType=sfix(16)  OutScaling=2^0
  TriGtr1 : Subsystem  mask(TriGtr){T=T, Td=Td}
      mask prompts: T "Period Time"; Td "Time Delay"
      mask help: Triangular Wave Generator with variable time delay
  Out1 : Outport
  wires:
  Sum/1 -> Out1/1
  Ampl./1 -> Sum/1
  TriGtr1/1(O) -> Ampl./1
  Offset/1 -> Sum/2

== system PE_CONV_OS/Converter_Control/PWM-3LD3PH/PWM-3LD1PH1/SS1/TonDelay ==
  s1 : Inport  Orientation=down  OutDataType=sfix(16)  OutScaling=2^0
  Int : Integrator  ExternalReset=falling
  Rel1 : Relay  OnSwitchValue=DT  OutDataType=sfix(16)  OutScaling=2^0
  s1d : Outport  InitialOutput=0
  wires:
  Rel1/1 -> s1d/1
  s1/1 -> Int/1, Int/2
  Int/1 -> Rel1/1

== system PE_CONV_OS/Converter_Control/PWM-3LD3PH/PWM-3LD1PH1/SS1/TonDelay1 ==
  s1 : Inport  Orientation=down  OutDataType=sfix(16)  OutScaling=2^0
  Int : Integrator  ExternalReset=falling
  Rel1 : Relay  OnSwitchValue=DT  OutDataType=sfix(16)  OutScaling=2^0
  s1d : Outport  InitialOutput=0
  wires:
  Rel1/1 -> s1d/1
  s1/1 -> Int/1, Int/2
  Int/1 -> Rel1/1

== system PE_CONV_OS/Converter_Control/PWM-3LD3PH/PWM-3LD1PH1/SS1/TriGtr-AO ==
  Ampl. : Gain  Gain=A  ParameterDataType=sfix(16)  ParameterScaling=2^0  OutDataType=sfix(16)  OutScaling=2^0
  Offset : Constant  Value=O  OutDataType=sfix(16)  OutScaling=2^0
  Sum : Sum  OutDataType=sfix(16)  OutScaling=2^0
  TriGtr1 : Subsystem  mask(TriGtr){T=T, Td=Td}
      mask prompts: T "Period Time"; Td "Time Delay"
      mask help: Triangular Wave Generator with variable time delay
  Out1 : Outport
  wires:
  Offset/1 -> Sum/2
  TriGtr1/1(O) -> Ampl./1
  Ampl./1 -> Sum/1
  Sum/1 -> Out1/1

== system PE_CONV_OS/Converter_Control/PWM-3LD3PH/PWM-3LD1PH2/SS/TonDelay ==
  s1 : Inport  Orientation=down  OutDataType=sfix(16)  OutScaling=2^0
  Int : Integrator  ExternalReset=falling
  Rel1 : Relay  OnSwitchValue=DT  OutDataType=sfix(16)  OutScaling=2^0
  s1d : Outport  InitialOutput=0
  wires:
  Int/1 -> Rel1/1
  s1/1 -> Int/2, Int/1
  Rel1/1 -> s1d/1

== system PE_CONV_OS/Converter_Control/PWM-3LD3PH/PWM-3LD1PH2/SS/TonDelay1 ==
  s1 : Inport  Orientation=down  OutDataType=sfix(16)  OutScaling=2^0
  Int : Integrator  ExternalReset=falling
  Rel1 : Relay  OnSwitchValue=DT  OutDataType=sfix(16)  OutScaling=2^0
  s1d : Outport  InitialOutput=0
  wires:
  Int/1 -> Rel1/1
  s1/1 -> Int/2, Int/1
  Rel1/1 -> s1d/1

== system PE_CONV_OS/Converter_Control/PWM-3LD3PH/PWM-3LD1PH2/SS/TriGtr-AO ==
  Ampl. : Gain  Gain=A  ParameterDataType=sfix(16)  ParameterScaling=2^0  OutDataType=sfix(16)  OutScaling=2^0
  Offset : Constant  Value=O  OutDataType=sfix(16)  OutScaling=2^0
  Sum : Sum  OutDataType=sfix(16)  OutScaling=2^0
  TriGtr1 : Subsystem  mask(TriGtr){T=T, Td=Td}
      mask prompts: T "Period Time"; Td "Time Delay"
      mask help: Triangular Wave Generator with variable time delay
  Out1 : Outport
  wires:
  Offset/1 -> Sum/2
  TriGtr1/1(O) -> Ampl./1
  Ampl./1 -> Sum/1
  Sum/1 -> Out1/1

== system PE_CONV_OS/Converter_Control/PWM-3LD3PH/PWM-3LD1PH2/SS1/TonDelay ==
  s1 : Inport  Orientation=down  OutDataType=sfix(16)  OutScaling=2^0
  Int : Integrator  ExternalReset=falling
  Rel1 : Relay  OnSwitchValue=DT  OutDataType=sfix(16)  OutScaling=2^0
  s1d : Outport  InitialOutput=0
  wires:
  Int/1 -> Rel1/1
  s1/1 -> Int/2, Int/1
  Rel1/1 -> s1d/1

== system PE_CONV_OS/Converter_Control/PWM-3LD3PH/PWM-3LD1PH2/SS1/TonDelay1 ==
  s1 : Inport  Orientation=down  OutDataType=sfix(16)  OutScaling=2^0
  Int : Integrator  ExternalReset=falling
  Rel1 : Relay  OnSwitchValue=DT  OutDataType=sfix(16)  OutScaling=2^0
  s1d : Outport  InitialOutput=0
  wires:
  Int/1 -> Rel1/1
  s1/1 -> Int/2, Int/1
  Rel1/1 -> s1d/1

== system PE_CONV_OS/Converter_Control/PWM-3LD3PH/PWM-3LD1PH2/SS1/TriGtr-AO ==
  Ampl. : Gain  Gain=A  ParameterDataType=sfix(16)  ParameterScaling=2^0  OutDataType=sfix(16)  OutScaling=2^0
  Offset : Constant  Value=O  OutDataType=sfix(16)  OutScaling=2^0
  Sum : Sum  OutDataType=sfix(16)  OutScaling=2^0
  TriGtr1 : Subsystem  mask(TriGtr){T=T, Td=Td}
      mask prompts: T "Period Time"; Td "Time Delay"
      mask help: Triangular Wave Generator with variable time delay
  Out1 : Outport
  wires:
  Sum/1 -> Out1/1
  Ampl./1 -> Sum/1
  TriGtr1/1(O) -> Ampl./1
  Offset/1 -> Sum/2

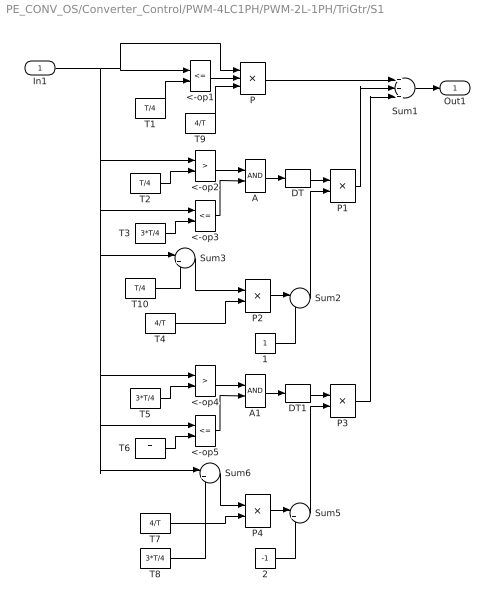
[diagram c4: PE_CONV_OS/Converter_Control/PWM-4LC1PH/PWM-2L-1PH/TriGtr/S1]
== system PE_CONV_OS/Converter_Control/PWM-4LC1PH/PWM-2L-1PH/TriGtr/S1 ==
  In1 : Inport  OutDataType=sfix(16)  OutScaling=2^0
  1 : Constant  OutDataType=sfix(16)  OutScaling=2^0
  2 : Constant  Value=-1  OutDataType=sfix(16)  OutScaling=2^0
  <-op1 : RelationalOperator  Operator=<=
  <-op2 : RelationalOperator  Operator=>
  <-op3 : RelationalOperator  Operator=<=
  <-op4 : RelationalOperator  Operator=>
  <-op5 : RelationalOperator  Operator=<=
  A : Logic  AllPortsSameDT=off
  A1 : Logic  AllPortsSameDT=off
  DT : DataTypeConversion
  DT1 : DataTypeConversion
  P : Product  Inputs=3  OutDataType=sfix(16)  OutScaling=2^0
  P{1..4} (4 alike) : Product  OutDataType=sfix(16)  OutScaling=2^0
  Sum1 : Sum  Inputs=+++  OutDataType=sfix(16)  OutScaling=2^0
  Sum2 : Sum  Inputs=|-+  OutDataType=sfix(16)  OutScaling=2^0
  Sum3 : Sum  Inputs=|+-  OutDataType=sfix(16)  OutScaling=2^0
  Sum5 : Sum  Inputs=|++  OutDataType=sfix(16)  OutScaling=2^0
  Sum6 : Sum  Inputs=|+-  OutDataType=sfix(16)  OutScaling=2^0
  T1 : Constant  Value=T/4  OutDataType=sfix(16)  OutScaling=2^0
  T10 : Constant  Value=T/4  OutDataType=sfix(16)  OutScaling=2^0
  T2 : Constant  Value=T/4  OutDataType=sfix(16)  OutScaling=2^0
  T3 : Constant  Value=3*T/4  OutDataType=sfix(16)  OutScaling=2^0
  T4 : Constant  Value=4/T  OutDataType=sfix(16)  OutScaling=2^0
  T5 : Constant  Value=3*T/4  OutDataType=sfix(16)  OutScaling=2^0
  T6 : Constant  Value=T  OutDataType=sfix(16)  OutScaling=2^0
  T7 : Constant  Value=4/T  OutDataType=sfix(16)  OutScaling=2^0
  T8 : Constant  Value=3*T/4  OutDataType=sfix(16)  OutScaling=2^0
  T9 : Constant  Value=4/T  OutDataType=sfix(16)  OutScaling=2^0
  Out1 : Outport
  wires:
  T10/1 -> Sum3/2
  T9/1 -> P/3
  DT1/1 -> P3/1
  DT/1 -> P1/1
  T1/1 -> <-op1/2
  <-op1/1 -> P/2
  P/1 -> Sum1/1
  T2/1 -> <-op2/2
  <-op2/1 -> A/1
  T3/1 -> <-op3/2
  <-op3/1 -> A/2
  A/1 -> DT/1
  T4/1 -> P2/2
  Sum3/1 -> P2/1
  In1/1 -> <-op2/1, <-op3/1, Sum3/1, <-op4/1, <-op5/1, Sum6/1, <-op1/1, P/1
  P1/1 -> Sum1/2
  P2/1 -> Sum2/1
  1/1 -> Sum2/2
  Sum2/1 -> P1/2
  T5/1 -> <-op4/2
  <-op4/1 -> A1/1
  T6/1 -> <-op5/2
  <-op5/1 -> A1/2
  A1/1 -> DT1/1
  T7/1 -> P4/2
  Sum6/1 -> P4/1
  P4/1 -> Sum5/1
  2/1 -> Sum5/2
  Sum5/1 -> P3/2
  T8/1 -> Sum6/2
  P3/1 -> Sum1/3
  Sum1/1 -> Out1/1

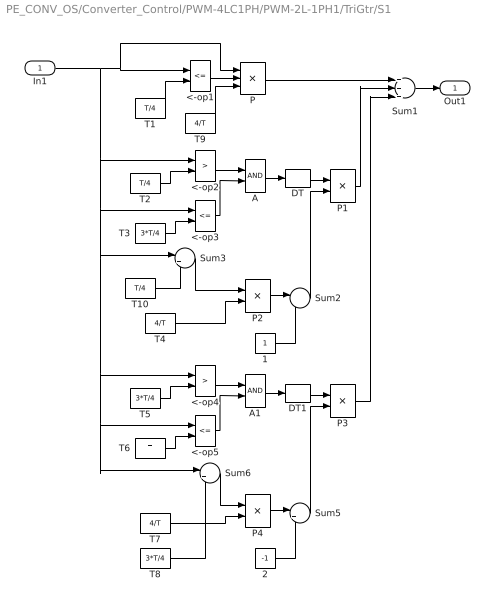
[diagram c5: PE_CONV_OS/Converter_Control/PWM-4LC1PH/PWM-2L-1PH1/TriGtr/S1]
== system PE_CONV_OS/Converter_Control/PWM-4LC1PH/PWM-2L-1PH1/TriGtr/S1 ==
  In1 : Inport  OutDataType=sfix(16)  OutScaling=2^0
  1 : Constant  OutDataType=sfix(16)  OutScaling=2^0
  2 : Constant  Value=-1  OutDataType=sfix(16)  OutScaling=2^0
  <-op1 : RelationalOperator  Operator=<=
  <-op2 : RelationalOperator  Operator=>
  <-op3 : RelationalOperator  Operator=<=
  <-op4 : RelationalOperator  Operator=>
  <-op5 : RelationalOperator  Operator=<=
  A : Logic  AllPortsSameDT=off
  A1 : Logic  AllPortsSameDT=off
  DT : DataTypeConversion
  DT1 : DataTypeConversion
  P : Product  Inputs=3  OutDataType=sfix(16)  OutScaling=2^0
  P{1..4} (4 alike) : Product  OutDataType=sfix(16)  OutScaling=2^0
  Sum1 : Sum  Inputs=+++  OutDataType=sfix(16)  OutScaling=2^0
  Sum2 : Sum  Inputs=|-+  OutDataType=sfix(16)  OutScaling=2^0
  Sum3 : Sum  Inputs=|+-  OutDataType=sfix(16)  OutScaling=2^0
  Sum5 : Sum  Inputs=|++  OutDataType=sfix(16)  OutScaling=2^0
  Sum6 : Sum  Inputs=|+-  OutDataType=sfix(16)  OutScaling=2^0
  T1 : Constant  Value=T/4  OutDataType=sfix(16)  OutScaling=2^0
  T10 : Constant  Value=T/4  OutDataType=sfix(16)  OutScaling=2^0
  T2 : Constant  Value=T/4  OutDataType=sfix(16)  OutScaling=2^0
  T3 : Constant  Value=3*T/4  OutDataType=sfix(16)  OutScaling=2^0
  T4 : Constant  Value=4/T  OutDataType=sfix(16)  OutScaling=2^0
  T5 : Constant  Value=3*T/4  OutDataType=sfix(16)  OutScaling=2^0
  T6 : Constant  Value=T  OutDataType=sfix(16)  OutScaling=2^0
  T7 : Constant  Value=4/T  OutDataType=sfix(16)  OutScaling=2^0
  T8 : Constant  Value=3*T/4  OutDataType=sfix(16)  OutScaling=2^0
  T9 : Constant  Value=4/T  OutDataType=sfix(16)  OutScaling=2^0
  Out1 : Outport
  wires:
  Sum1/1 -> Out1/1
  P3/1 -> Sum1/3
  T8/1 -> Sum6/2
  Sum5/1 -> P3/2
  2/1 -> Sum5/2
  P4/1 -> Sum5/1
  Sum6/1 -> P4/1
  T7/1 -> P4/2
  A1/1 -> DT1/1
  <-op5/1 -> A1/2
  T6/1 -> <-op5/2
  <-op4/1 -> A1/1
  T5/1 -> <-op4/2
  Sum2/1 -> P1/2
  1/1 -> Sum2/2
  P2/1 -> Sum2/1
  P1/1 -> Sum1/2
  In1/1 -> P/1, <-op1/1, Sum6/1, <-op5/1, <-op4/1, Sum3/1, <-op3/1, <-op2/1
  Sum3/1 -> P2/1
  T4/1 -> P2/2
  A/1 -> DT/1
  <-op3/1 -> A/2
  T3/1 -> <-op3/2
  <-op2/1 -> A/1
  T2/1 -> <-op2/2
  P/1 -> Sum1/1
  <-op1/1 -> P/2
  T1/1 -> <-op1/2
  DT/1 -> P1/1
  DT1/1 -> P3/1
  T9/1 -> P/3
  T10/1 -> Sum3/2
